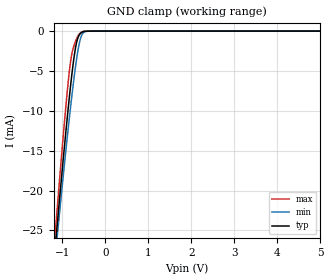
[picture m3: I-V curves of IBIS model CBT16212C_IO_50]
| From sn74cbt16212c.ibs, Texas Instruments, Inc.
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[Model]   CBT16212C_IO_50
Model_type  Terminator
| variable   typ   min   max
C_comp   8.63pF   6.53pF   14.30pF
| C_tri-state   8.63pF   6.53pF   14.30pF
[Temperature Range]   40   100   -40
| Ambient temperature   25   85   -40
[Voltage range]   5   4.5   5.5
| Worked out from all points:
|   GND clamp passes 1 mA (typ) near -0.65 V on its own axis
[GND Clamp]
| CBT16212C_IO_50
|   Voltage   I(typ)   I(min)   I(max)
-5V       -286.9mA   -267.5mA   -309.2mA
-1.19V    -28.47mA   -29.59mA   -26.88mA
-1.155V   -26.34mA   -27.64mA   -24.51mA
-1.12V    -24.23mA   -25.7mA    -22.17mA
-1.085V   -22.14mA   -23.78mA   -19.85mA
-925mV    -12.91mA   -15.26mA   -9.733mA
-815mV    -7.1mA     -9.758mA   -4.012mA
-760mV    -4.528mA   -7.198mA   -2.356mA
-675mV    -1.54mA    -3.676mA   -1.013mA
-610mV    -508.2uA   -1.614mA   -383.4uA
-545mV    -149.1uA   -459.7uA   -90.44uA
5V        665.2pA    1.972nA    257.8pA
